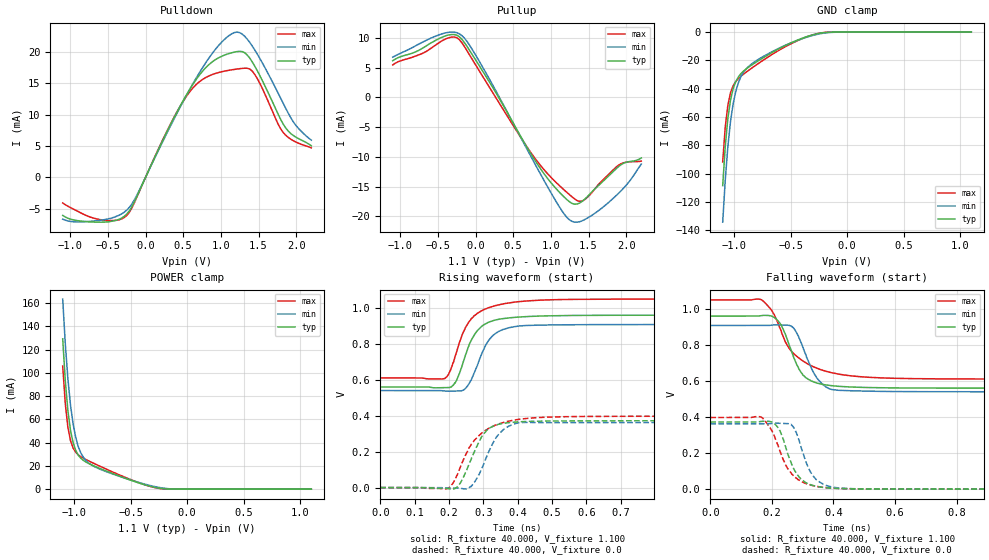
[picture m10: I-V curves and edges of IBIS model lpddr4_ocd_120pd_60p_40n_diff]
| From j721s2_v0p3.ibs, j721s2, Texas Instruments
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|   Model lpddr4_ocd_120pd_60p_40n_diff
[Model] lpddr4_ocd_120pd_60p_40n_diff
Model_type I/O
Polarity   Non-Inverting
Enable   Active-High
Vinl =  0.113V
Vinh =  0.253V
Vmeas =  0.183V
C_comp   1.509pF   1.327pF   1.810pF
[Model Spec]
Vinh   0.253V   0.247V   0.265V
Vinl   0.113V   0.107V   0.125V
Vmeas   0.183V   0.176V   0.195V
[Temperature Range]   25.000   0.125k   -40.000
[Voltage Range]   1.100V   1.060V   1.170V
[Pullup Reference]   1.100V   1.060V   1.170V
[Pulldown Reference]   0.0V   0.0V   0.0V
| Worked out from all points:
|   slope of the pulldown table from 0 to 0.165 V, typ, clamps not added: 38.6 ohm
|   slope of the pullup table from 0 to 0.165 V, typ, clamps not added: 49.3 ohm
|   GND clamp passes 1 mA (typ) near -0.25 V on its own axis
|   POWER clamp passes 1 mA (typ) near -0.26 V on its own axis
|   rising waveform, R_fixture 40.000, V_fixture 1.100: 20-80 % time 54.3ps typ, 54.2ps min, 64.3ps max; typ from 0.56 V to 0.96 V
|   rising waveform, R_fixture 40.000, V_fixture 0.0: 20-80 % time 54.9ps typ, 54.7ps min, 79.8ps max; typ from 0 V to 0.372 V
|   falling waveform, R_fixture 40.000, V_fixture 1.100: 20-80 % time 60ps typ, 57.9ps min, 104ps max; typ from 0.96 V to 0.56 V
|   falling waveform, R_fixture 40.000, V_fixture 0.0: 20-80 % time 52.9ps typ, 50ps min, 65.6ps max; typ from 0.372 V to 0 V
[Pulldown]
|Voltage   I(typ)   I(min)   I(max)
-1.1V     -6.056mA   -6.655mA   -4.075mA
-658mV    -7.127mA   -6.914mA   -6.587mA
-284mV    -6.208mA   -5.549mA   -6.391mA
-113mV    -2.983mA   -2.787mA   -3.073mA
295mV     7.517mA    7.322mA    7.635mA
567mV     13.62mA    13.58mA    13.31mA
839mV     17.92mA    18.95mA    16.13mA
1.179V    19.93mA    23.04mA    17.18mA
1.418V    18.32mA    20.86mA    16.88mA
1.826V    8.488mA    11.79mA    7.151mA
1.996V    6.386mA    8.257mA    5.615mA
2.2V      5.031mA    5.921mA    4.7mA
[Pullup]
|Voltage   I(typ)   I(min)   I(max)
-1.1V     6.194mA    6.785mA    5.476mA
-352mV    10.54mA    10.98mA    10.07mA
-249mV    10.48mA    10.91mA    10.07mA
-181mV    9.79mA     10.42mA    9.201mA
125mV     3.816mA    4.426mA    2.927mA
771mV     -10.24mA   -10.78mA   -9.944mA
1.111V    -15.92mA   -18.38mA   -14.81mA
1.281V    -17.84mA   -20.86mA   -16.73mA
1.418V    -17.46mA   -20.74mA   -17.41mA
1.724V    -13.72mA   -18.12mA   -13.47mA
1.928V    -11.34mA   -15.74mA   -11.16mA
2.2V      -10.19mA   -11.2mA    -10.71mA
[GND_clamp]
|Voltage   I(typ)   I(min)   I(max)
-1.1V     -108.4mA   -134.2mA   -91.64mA
-1.077V   -80.17mA   -103.9mA   -66.63mA
-1.054V   -60.68mA   -80.47mA   -51.43mA
-1.031V   -48.01mA   -63.16mA   -42.83mA
-1.008V   -40.05mA   -50.75mA   -37.96mA
-985mV    -35.04mA   -42.04mA   -34.98mA
-940mV    -29.42mA   -31.64mA   -31.22mA
-894mV    -26.11mA   -26.16mA   -28.35mA
-848mV    -23.5mA    -22.73mA   -25.7mA
-527mV    -8.739mA   -8.686mA   -9.514mA
-229mV    -630.6uA   -1.042mA   -565.6uA
1.1V      0A         0A         0A
[POWER_clamp]
|Voltage   I(typ)   I(min)   I(max)
-1.1V     129.2mA    163.4mA    105.9mA
-1.077V   92.86mA    124.8mA    73.4mA
-1.054V   67.3mA     94.73mA    53.17mA
-1.031V   50.48mA    72.25mA    41.67mA
-1.008V   39.92mA    56.03mA    35.37mA
-985mV    33.38mA    44.6mA     31.76mA
-963mV    29.31mA    36.69mA    29.53mA
-917mV    24.75mA    27.38mA    26.61mA
-871mV    22.09mA    22.57mA    24.31mA
-619mV    11.98mA    11.76mA    13.12mA
-229mV    602.6uA    1.183mA    400.7uA
1.1V      0A         0A         0A
[Ramp]
| variable   typ   min   max
dV/dt_r   0.223/54.399p   0.217/54.465p   0.238/80.305p
dV/dt_f   0.240/59.185p   0.221/57.521p   0.264/0.103n
R_load = 40.000
[Rising Waveform]
R_fixture= 40.000
V_fixture= 1.100
V_fixture_min= 1.060
V_fixture_max= 1.170
|time   V(typ)   V(min)   V(max)
0s        560.1mV    540.2mV    610.4mV
188ps     556.3mV    537.6mV    607.3mV
199ps     556.5mV    536.4mV    630.9mV
218ps     582.6mV    537.4mV    732.1mV
239ps     683.4mV    540.2mV    854mV
262ps     809.8mV    591.7mV    931.4mV
297ps     900.8mV    753.1mV    986.1mV
341ps     935.5mV    865.3mV    1.015V
422ps     951.5mV    902.1mV    1.038V
3ns       959.7mV    907.8mV    1.049V
[Rising Waveform]
R_fixture= 40.000
V_fixture= 0.0
V_fixture_min= 0.0
V_fixture_max= 0.0
|time   V(typ)   V(min)   V(max)
0s        169.1uV    276.9uV    327.4uV
197ps     -4.865mV   -3.346mV   -4.438mV
226ps     5.917mV    -2.537mV   79.43mV
254ps     110.2mV    -6.15mV    203.3mV
281ps     228.6mV    50.18mV    277.2mV
316ps     329.6mV    201.1mV    330mV
338ps     348.7mV    281mV      349.6mV
362ps     359.3mV    328.6mV    364.4mV
443ps     369.1mV    362.2mV    387.9mV
3ns       372.4mV    362.5mV    397.6mV
[Falling Waveform]
R_fixture= 40.000
V_fixture= 1.100
V_fixture_min= 1.060
V_fixture_max= 1.170
|time   V(typ)   V(min)   V(max)
0s        959.7mV    907.8mV    1.049V
167ps     963.5mV    907.8mV    1.05V
218ps     937.9mV    911.2mV    927.9mV
261ps     778.8mV    906.1mV    769.8mV
300ps     634.3mV    789.1mV    712mV
330ps     599mV      664.3mV    683mV
360ps     582.9mV    589.1mV    662.3mV
394ps     574mV      552.7mV    646mV
475ps     565.5mV    545.1mV    625.5mV
3ns       560.1mV    540.2mV    610.4mV
[Falling Waveform]
R_fixture= 40.000
V_fixture= 0.0
V_fixture_min= 0.0
V_fixture_max= 0.0
|time   V(typ)   V(min)   V(max)
0s        372.4mV    362.5mV    397.6mV
167ps     376.2mV    362.5mV    398.6mV
199ps     372.8mV    364.3mV    327.9mV
219ps     343.5mV    365.9mV    247.7mV
244ps     238mV      364.7mV    136.7mV
262ps     149.4mV    359.3mV    91.09mV
288ps     67.87mV    273.7mV    50.48mV
325ps     24.47mV    96.29mV    22.91mV
384ps     6.944mV    17.23mV    7.323mV
3ns       167.8uV    276.2uV    327uV
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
